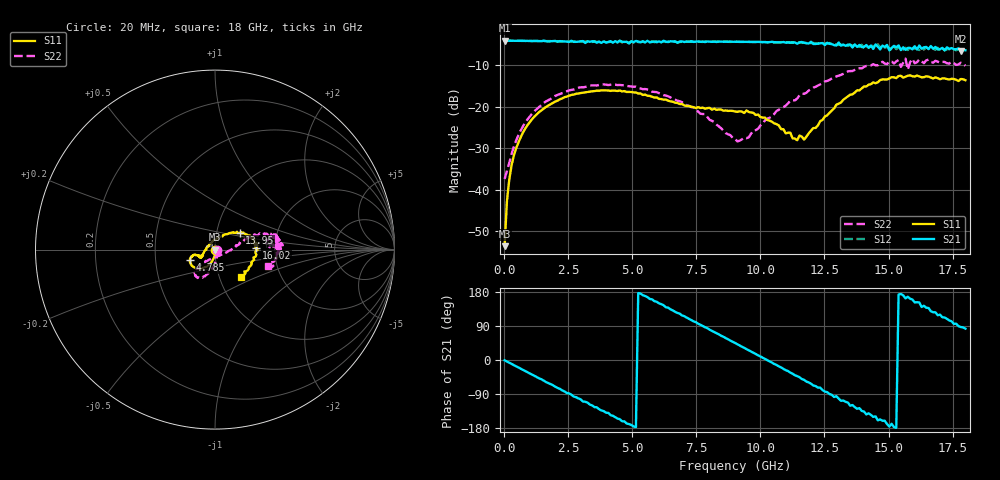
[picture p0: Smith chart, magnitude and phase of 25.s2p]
!Agilent Technologies,N5230A,US43500223,A.07.50.48
!Agilent N5230A: A.07.50.48
!Date: Sunday, January 10, 2016 12:09:51
!Correction: S11(Full 2 Port(1,2))
!S21(Full 2 Port(1,2))
!S12(Full 2 Port(1,2))
!S22(Full 2 Port(1,2))
!S2P File: Measurements: S11, S21, S12, S22:
# Hz S  RI  R 50
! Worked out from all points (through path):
!   201 points, 20 MHz to 18 GHz, reference 50 ohm
!   highest |S21| = -4.12 dB at 20 MHz (marker M1); lowest = -6.7 dB at 17.82 GHz (marker M2)
!   group delay of S21, straight-line fit = 98.5 ps
!   lowest |S11| = -53.5 dB at 20 MHz (marker M3), VSWR 1.00, Z = 50.2 - j0.124 ohm
!   |S11| at or under -10 dB: start of sweep to end of sweep
!   |S22| runs from -37.4 to -8.4 dB; largest |S21 - S12| = 0.086
!   S11 on the Smith chart (normalised r, x): 20 MHz: 1.00, -0.00; 4.785 GHz: 0.75, -0.09; 13.95 GHz: 1.29, +0.25; 16.02 GHz: 1.60, +0.04; 18 GHz: 1.27, -0.40
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2e7  0.0017 -0.00123  0.6223 -0.0084  0.6221 -0.00819  0.0135 -0.000781
1.099e8  0.00221 -0.00692  0.6207 -0.043  0.6196 -0.0431  0.0144 -0.00864
2.897e8  0.00144 -0.0196  0.6104 -0.1115  0.6103 -0.1121  0.0134 -0.0233
7.392e8  -0.00741 -0.0486  0.556 -0.2742  0.5555 -0.2748  0.00611 -0.0582
1.9978e9  -0.0583 -0.0996  0.2064 -0.5821  0.2059 -0.5818  -0.0356 -0.1305
3.0766e9  -0.1051 -0.1032  -0.2061 -0.5814  -0.1945 -0.5775  -0.0725 -0.155
4.7847e9  -0.1381 -0.0597  -0.5911 -0.1292  -0.5901 -0.1153  -0.1095 -0.1408
6.0433e9  -0.1206 -0.0306  -0.5272 0.3089  -0.5151 0.3223  -0.1005 -0.1055
7.5716e9  -0.0922 -0.0358  -0.0612 0.607  -0.0522 0.6029  -0.0549 -0.0681
9.01e9  -0.0768 -0.0422  0.4272 0.4281  0.4361 0.4187  0.00823 -0.0404
1.04484e10  -0.0635 -0.0181  0.599 -0.0706  0.5888 -0.0862  0.0762 -0.00706
1.14373e10  -0.0345 0.0195  0.4211 -0.3869  0.4245 -0.4069  0.1234 0.0229
1.20666e10  -0.000255 0.0555  0.2195 -0.5245  0.228 -0.5385  0.1611 0.0518
1.30555e10  0.0668 0.0858  -0.1222 -0.5792  -0.1251 -0.5393  0.2207 0.0851
1.39545e10  0.1376 0.0934  -0.3656 -0.373  -0.3974 -0.3894  0.2755 0.088
1.44939e10  0.1741 0.0796  -0.4807 -0.2907  -0.4449 -0.2435  0.3075 0.0689
1.50333e10  0.2097 0.0617  -0.4758 -0.0366  -0.5088 -0.0416  0.3454 0.0673
1.51232e10  0.22 0.0548  -0.4988 -0.1027  -0.4788 -0.0369  0.3473 0.0304
1.60222e10  0.2303 0.0112  -0.4713 0.2508  -0.4552 0.2093  0.3329 0.0217
1.69212e10  0.2117 -0.0617  -0.2309 0.4306  -0.2394 0.4513  0.3464 -0.0332
1.78202e10  0.17 -0.1324  0.0233 0.4644  0.04 0.4676  0.3251 -0.092
1.8e10  0.1441 -0.1503  0.0594 0.4748  0.0899 0.4694  0.2978 -0.09
